(* Logix 5000 AddOnInstructionDefinition export AMCI_SD4840E2_Enable_Driver; software revision 20.03 *)

ADD_ON_INSTRUCTION AMCI_SD4840E2_Enable_Driver   (* revision 1.0, vendor AMCI *)
VAR_IN_OUT
   AMCI_SD4840E2_output_data : _000A:SD4840E2_4342D302:O:0; {required}
END_VAR
VAR
   command_data_block : INT[10];
        [0]   // Command Bits MSW
        [1]   // Command Bits LSW
        [2]   // Upper Target Position
        [3]   // Lower Target Position
        [4]   // Upper Programmed Speed
        [5]   // Lower Programmed Speed
END_VAR

ROUTINE Logic   (* ladder *)
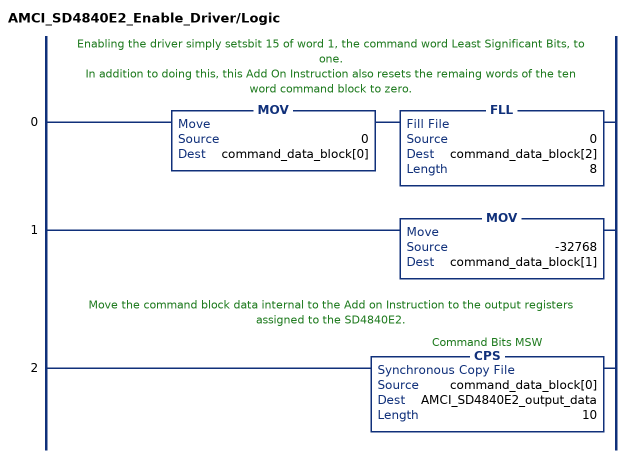
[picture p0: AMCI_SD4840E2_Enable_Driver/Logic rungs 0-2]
   // Enabling the driver simply setsbit 15 of word 1, the command word Least Significant Bits, to one.
   // In addition to doing this, this Add On Instruction also resets the remaing words of the ten word command block to zero.
   0: MOV(0,command_data_block[0])FLL(0,command_data_block[2],8);
   1: MOV(-32768,command_data_block[1]);
   // Move the command block data internal to the Add on Instruction to the output registers assigned to the SD4840E2.
   2: CPS(command_data_block[0],AMCI_SD4840E2_output_data,10);
END_ROUTINE
END_ADD_ON_INSTRUCTION
